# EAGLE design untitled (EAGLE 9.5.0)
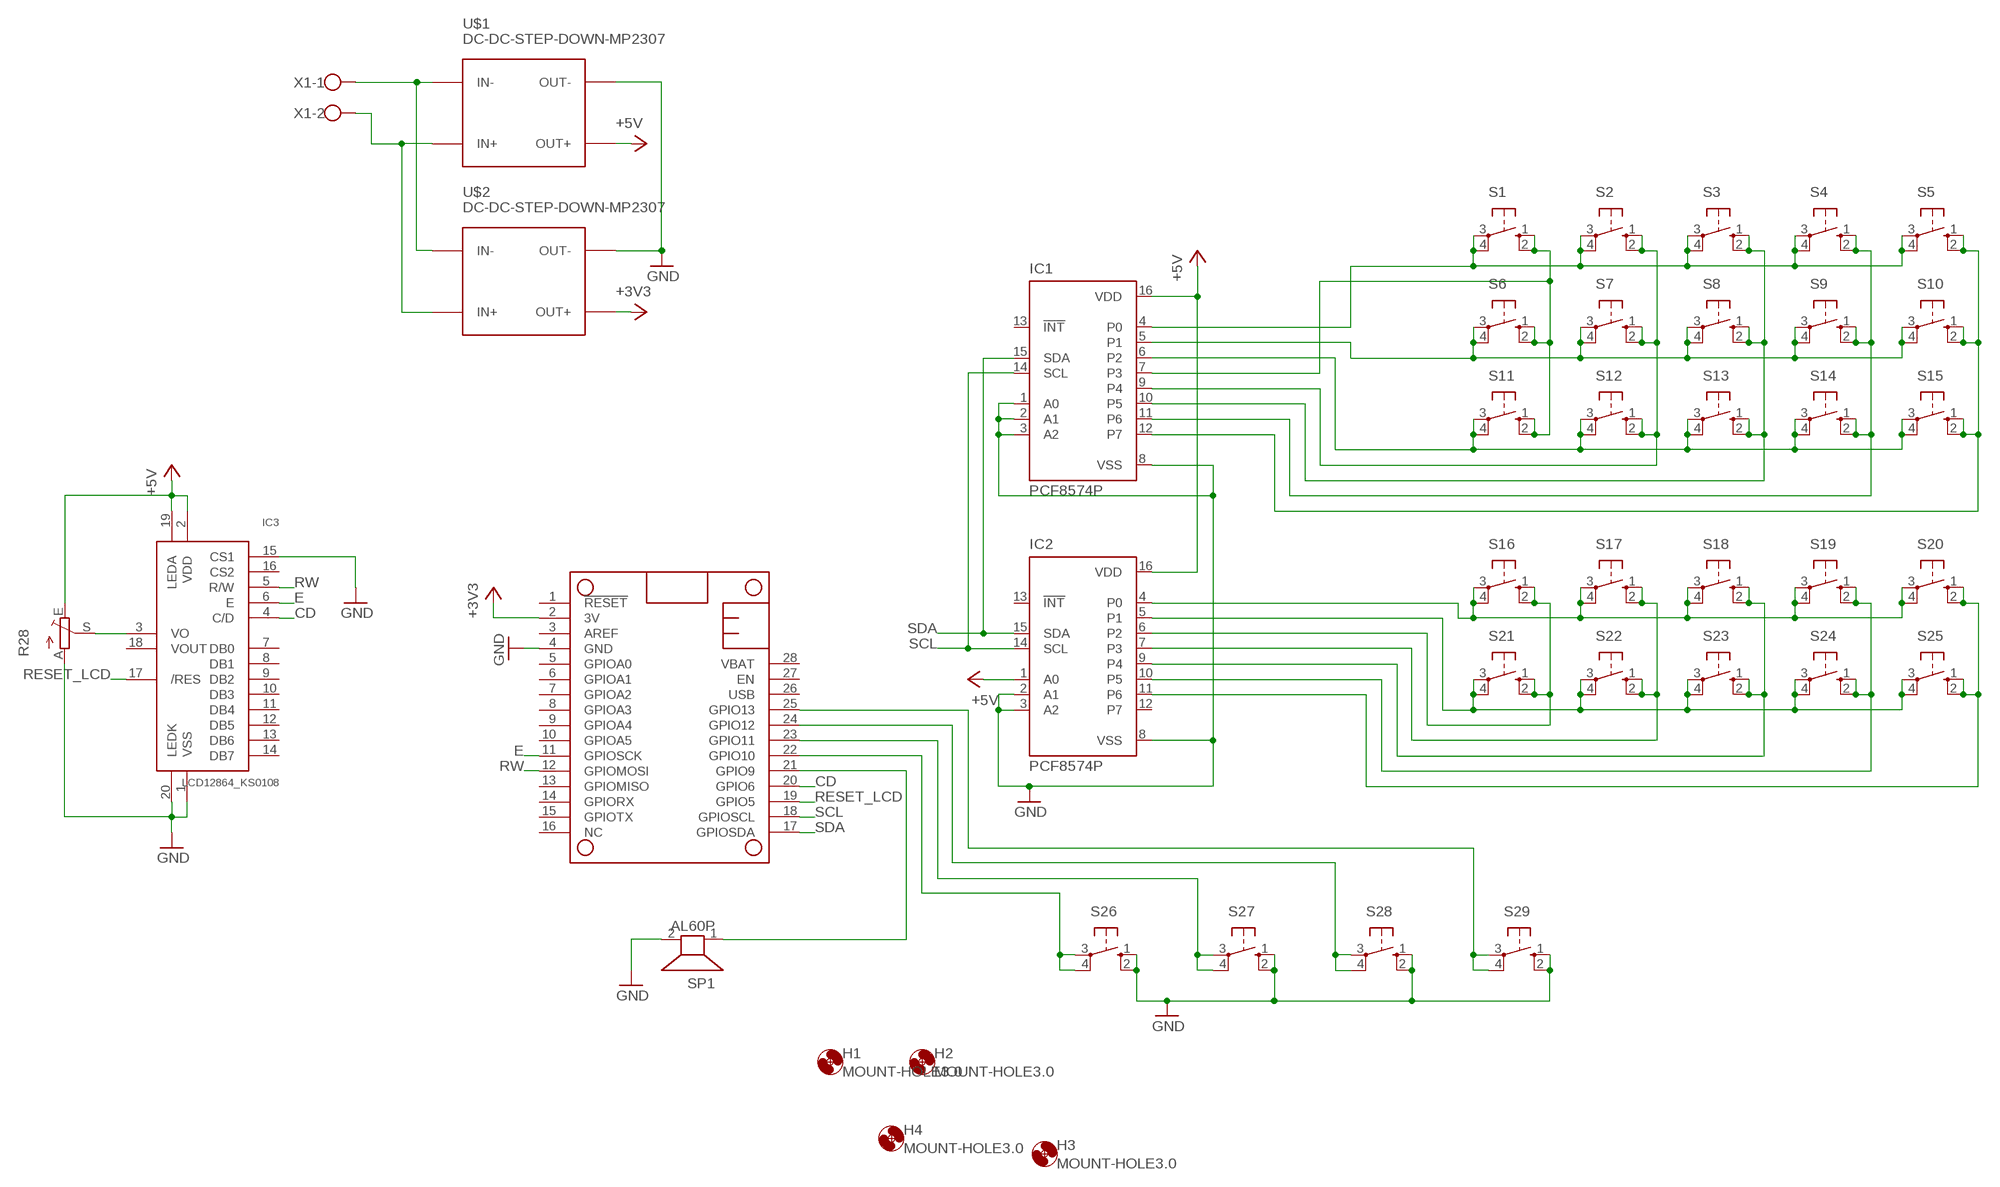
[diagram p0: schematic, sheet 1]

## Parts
H1  MOUNT-HOLE3.0  [3,0]
H2  MOUNT-HOLE3.0  [3,0]
H3  MOUNT-HOLE3.0  [3,0]
H4  MOUNT-HOLE3.0  [3,0]
IC1  PCF8574P  [DIL16]
IC2  PCF8574P  [DIL16]
IC3  LCD12864_KS0108  [RG12864]
MS1  FEATHERWING  [FEATHERWING]
R28  TRIM_EU-LI10  [LI10]
S1  10-XX  [B3F-10XX]
S2  10-XX  [B3F-10XX]
S3  10-XX  [B3F-10XX]
S4  10-XX  [B3F-10XX]
S5  10-XX  [B3F-10XX]
S6  10-XX  [B3F-10XX]
S7  10-XX  [B3F-10XX]
S8  10-XX  [B3F-10XX]
S9  10-XX  [B3F-10XX]
S10  10-XX  [B3F-10XX]
S11  10-XX  [B3F-10XX]
S12  10-XX  [B3F-10XX]
S13  10-XX  [B3F-10XX]
S14  10-XX  [B3F-10XX]
S15  10-XX  [B3F-10XX]
S16  10-XX  [B3F-10XX]
S17  10-XX  [B3F-10XX]
S18  10-XX  [B3F-10XX]
S19  10-XX  [B3F-10XX]
S20  10-XX  [B3F-10XX]
S21  10-XX  [B3F-10XX]
S22  10-XX  [B3F-10XX]
S23  10-XX  [B3F-10XX]
S24  10-XX  [B3F-10XX]
S25  10-XX  [B3F-10XX]
S26  10-XX  [B3F-10XX]
S27  10-XX  [B3F-10XX]
S28  10-XX  [B3F-10XX]
S29  10-XX  [B3F-10XX]
SP1  AL60P  [AL60P]
U$1  DC-DC-STEP-DOWN-MP2307  [DC-DC-STEP-DOWN-MP2307]
U$2  DC-DC-STEP-DOWN-MP2307  [DC-DC-STEP-DOWN-MP2307]
X1  W237-102  [W237-102]

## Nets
3V: MS1.2(3V) ; supply symbol labelled +3V3
+3V3: U$2.OUT+
+5V: IC1.16(VDD) IC2.1(A0) IC2.16(VDD) IC3.2(VDD) IC3.19(LEDA) R28.E U$1.OUT+
CD: IC3.4(C/D) MS1.20(GPIO6)
E: IC3.6(E) MS1.11(GPIOSCK)
GND: IC1.1(A0) IC1.2(A1) IC1.3(A2) IC1.8(VSS) IC2.2(A1) IC2.3(A2) IC2.8(VSS) IC3.1(VSS) IC3.15(CS1) IC3.20(LEDK) MS1.4(GND) R28.A S26.1(S) S26.2(S1) S27.1(S) S27.2(S1) S28.1(S) S28.2(S1) S29.1(S) S29.2(S1) SP1.2 U$1.OUT- U$2.OUT-
N$1: IC1.4(P0) S1.3(P) S1.4(P1) S2.3(P) S2.4(P1) S3.3(P) S3.4(P1) S4.3(P) S4.4(P1) S5.3(P) S5.4(P1)
N$3: IC1.5(P1) S6.3(P) S6.4(P1) S7.3(P) S7.4(P1) S8.3(P) S8.4(P1) S9.3(P) S9.4(P1) S10.3(P) S10.4(P1)
N$4: MS1.25(GPIO13) S29.3(P) S29.4(P1)
N$5: MS1.24(GPIO12) S28.3(P) S28.4(P1)
N$6: MS1.23(GPIO11) S27.3(P) S27.4(P1)
N$7: MS1.22(GPIO10) S26.3(P) S26.4(P1)
N$8: IC1.6(P2) S11.3(P) S11.4(P1) S12.3(P) S12.4(P1) S13.3(P) S13.4(P1) S14.3(P) S14.4(P1) S15.3(P) S15.4(P1)
N$9: IC1.7(P3) S1.1(S) S1.2(S1) S6.1(S) S6.2(S1) S11.1(S) S11.2(S1)
N$10: MS1.21(GPIO9) SP1.1
N$11: IC1.10(P5) S3.1(S) S3.2(S1) S8.1(S) S8.2(S1) S13.1(S) S13.2(S1)
N$12: IC1.11(P6) S4.1(S) S4.2(S1) S9.1(S) S9.2(S1) S14.1(S) S14.2(S1)
N$13: IC1.12(P7) S5.1(S) S5.2(S1) S10.1(S) S10.2(S1) S15.1(S) S15.2(S1)
N$16: U$1.IN- U$2.IN- X1.1
N$17: U$1.IN+ U$2.IN+ X1.2
N$21: IC1.9(P4) S2.1(S) S2.2(S1) S7.1(S) S7.2(S1) S12.1(S) S12.2(S1)
N$26: IC2.4(P0) S16.3(P) S16.4(P1) S17.3(P) S17.4(P1) S18.3(P) S18.4(P1) S19.3(P) S19.4(P1) S20.3(P) S20.4(P1)
N$28: IC2.7(P3) S17.1(S) S17.2(S1) S22.1(S) S22.2(S1)
N$29: IC2.5(P1) S21.3(P) S21.4(P1) S22.3(P) S22.4(P1) S23.3(P) S23.4(P1) S24.3(P) S24.4(P1) S25.3(P) S25.4(P1)
N$31: IC2.6(P2) S16.1(S) S16.2(S1) S21.1(S) S21.2(S1)
N$32: IC2.9(P4) S18.1(S) S18.2(S1) S23.1(S) S23.2(S1)
N$33: IC2.10(P5) S19.1(S) S19.2(S1) S24.1(S) S24.2(S1)
N$34: IC2.11(P6) S20.1(S) S20.2(S1) S25.1(S) S25.2(S1)
N$71: IC3.3(VO) R28.S
RESET_LCD: IC3.17(/RES) MS1.19(GPIO5)
RW: IC3.5(R/W) MS1.12(GPIOMOSI)
SCL: IC1.14(SCL) IC2.14(SCL) MS1.18(GPIOSCL)
SDA: IC1.15(SDA) IC2.15(SDA) MS1.17(GPIOSDA)
Unconnected: IC1.13(!INT) IC2.12(P7) IC2.13(!INT) IC3.7(DB0) IC3.8(DB1) IC3.9(DB2) IC3.10(DB3) IC3.11(DB4) IC3.12(DB5) IC3.13(DB6) IC3.14(DB7) IC3.16(CS2) IC3.18(VOUT) MS1.1(!RESET) MS1.3(AREF) MS1.5(GPIOA0) MS1.6(GPIOA1) MS1.7(GPIOA2) MS1.8(GPIOA3) MS1.9(GPIOA4) MS1.10(GPIOA5) MS1.13(GPIOMISO) MS1.14(GPIORX) MS1.15(GPIOTX) MS1.16(NC) MS1.26(USB) MS1.27(EN) MS1.28(VBAT)

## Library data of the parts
H1-H4 = holes:MOUNT-HOLE: MOUNTING HOLE with drill center marker
IC1 IC2 = micro-philips:PCF8574: I2C-Bus Remote 8-bit I/O expander http://www.semiconductors.philips.com/acrobat_download/datasheets/PCF8574_4.pdf
IC3 = DodoLcdR2:LCD12864_KS0108: LCD 128 x 64 controller KS0108
MS1 = adafruit:FEATHERWING
R28 = pot:TRIM_EU-: POTENTIOMETER
S1-S29 = switch-omron:10-XX: OMRON SWITCH; MPN: B3F-1000; OC_FARNELL: 176432; OC_NEWARK: 36M3542
SP1 = buzzer:AL60P: SPEAKER; OC_FARNELL: unknown; OC_NEWARK: unknown
U$1 U$2 = diy-modules:DC-DC-STEP-DOWN-MP2307: DC/DC Step-Down Regulator based on MP2307DN chip MP2307 datasheet available here: https://cdn-shop.adafruit.com/datasheets/MP2307_r1.9.pdf Click here to find device on ebay.com
X1 = con-wago-500:W237-102: WAGO SCREW CLAMP; MPN: 237-102; OC_FARNELL: unknown; OC_NEWARK: 70K9898

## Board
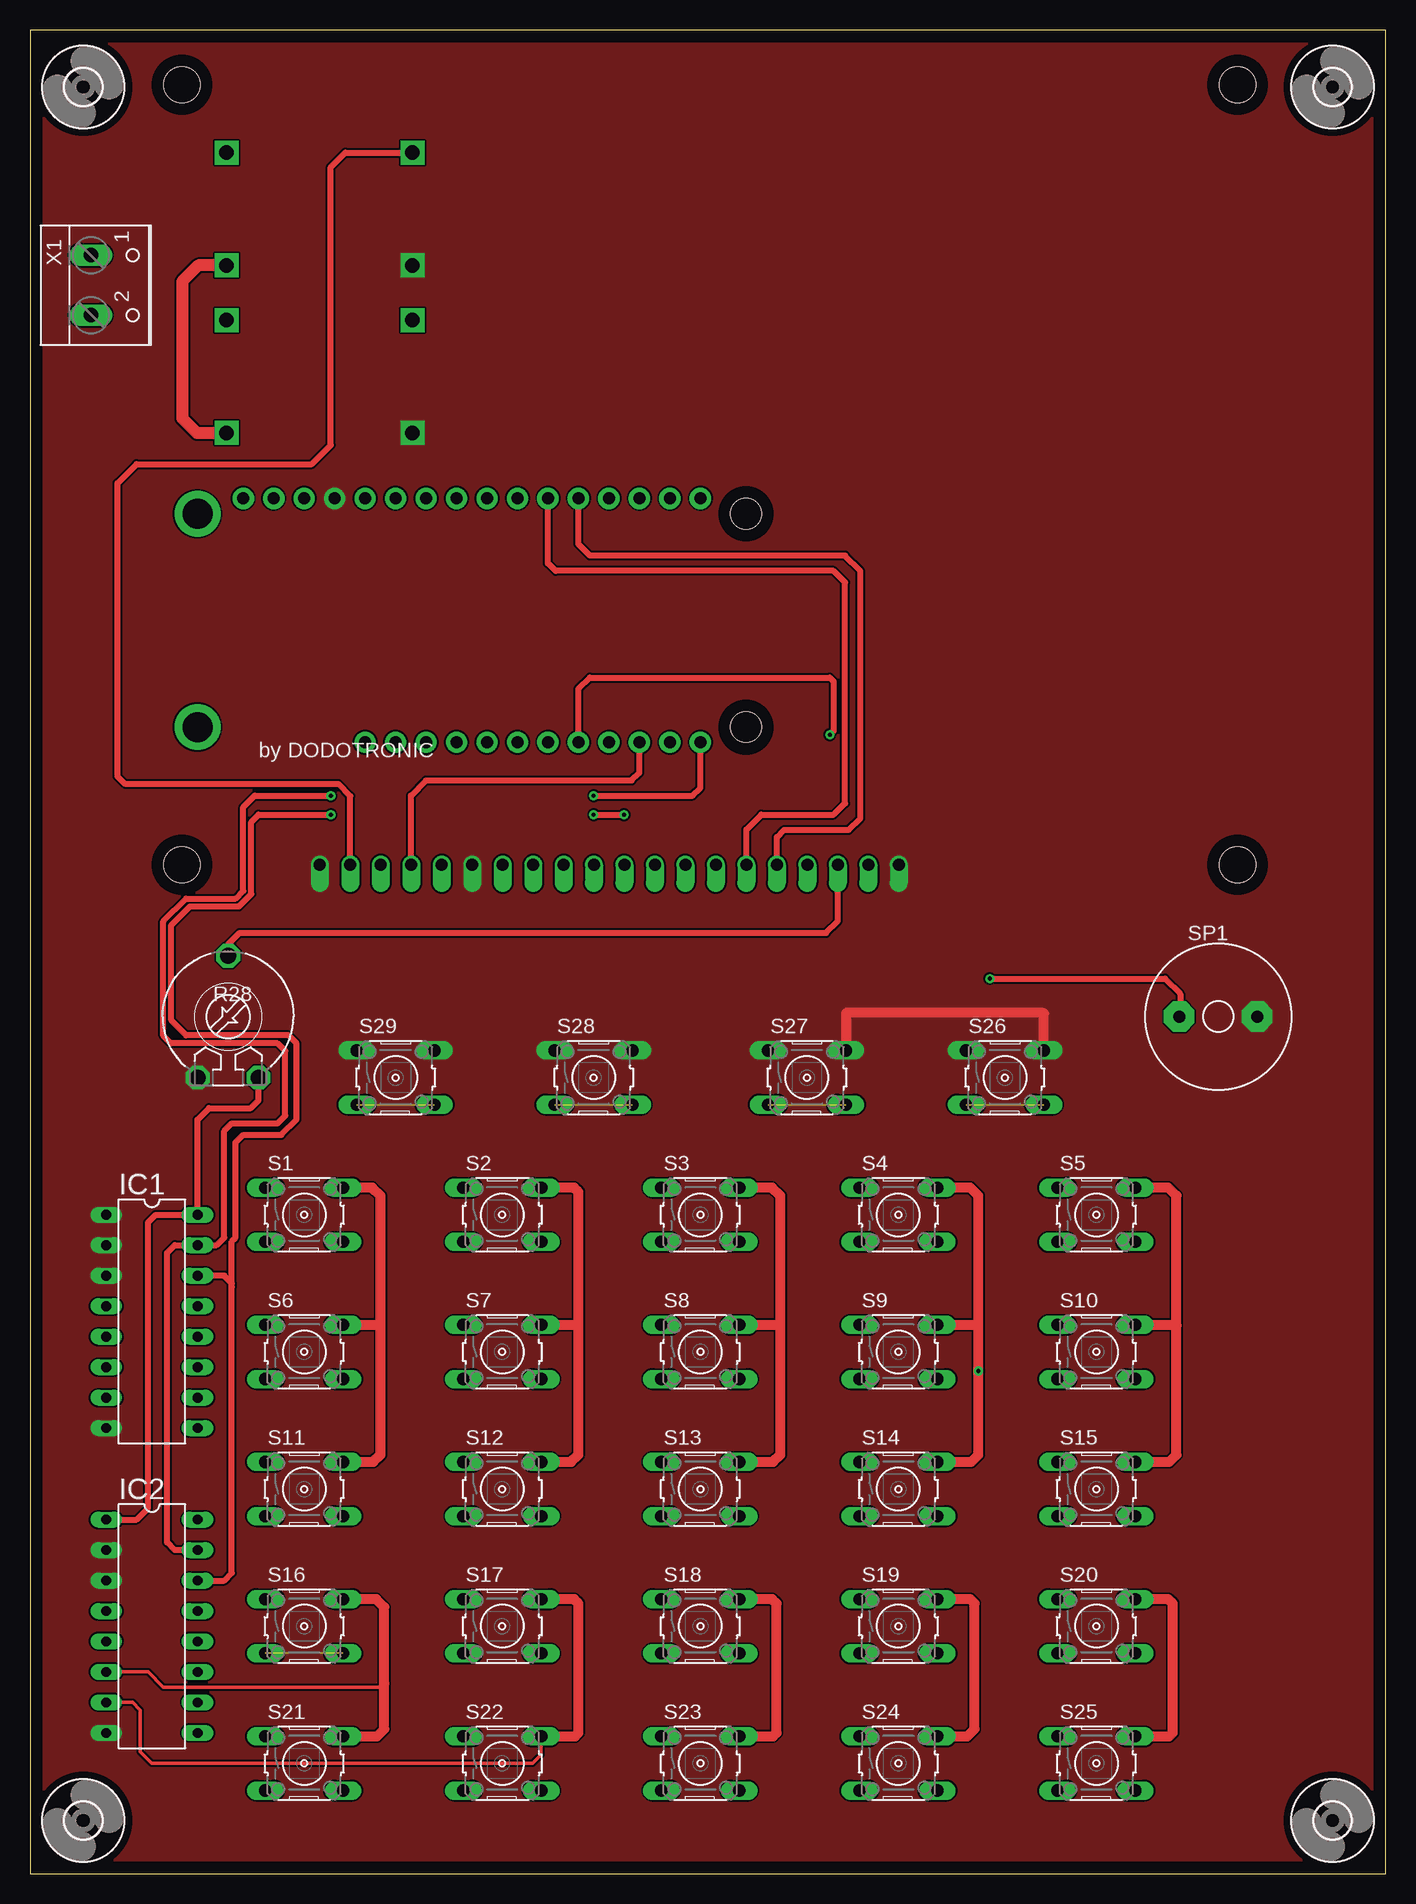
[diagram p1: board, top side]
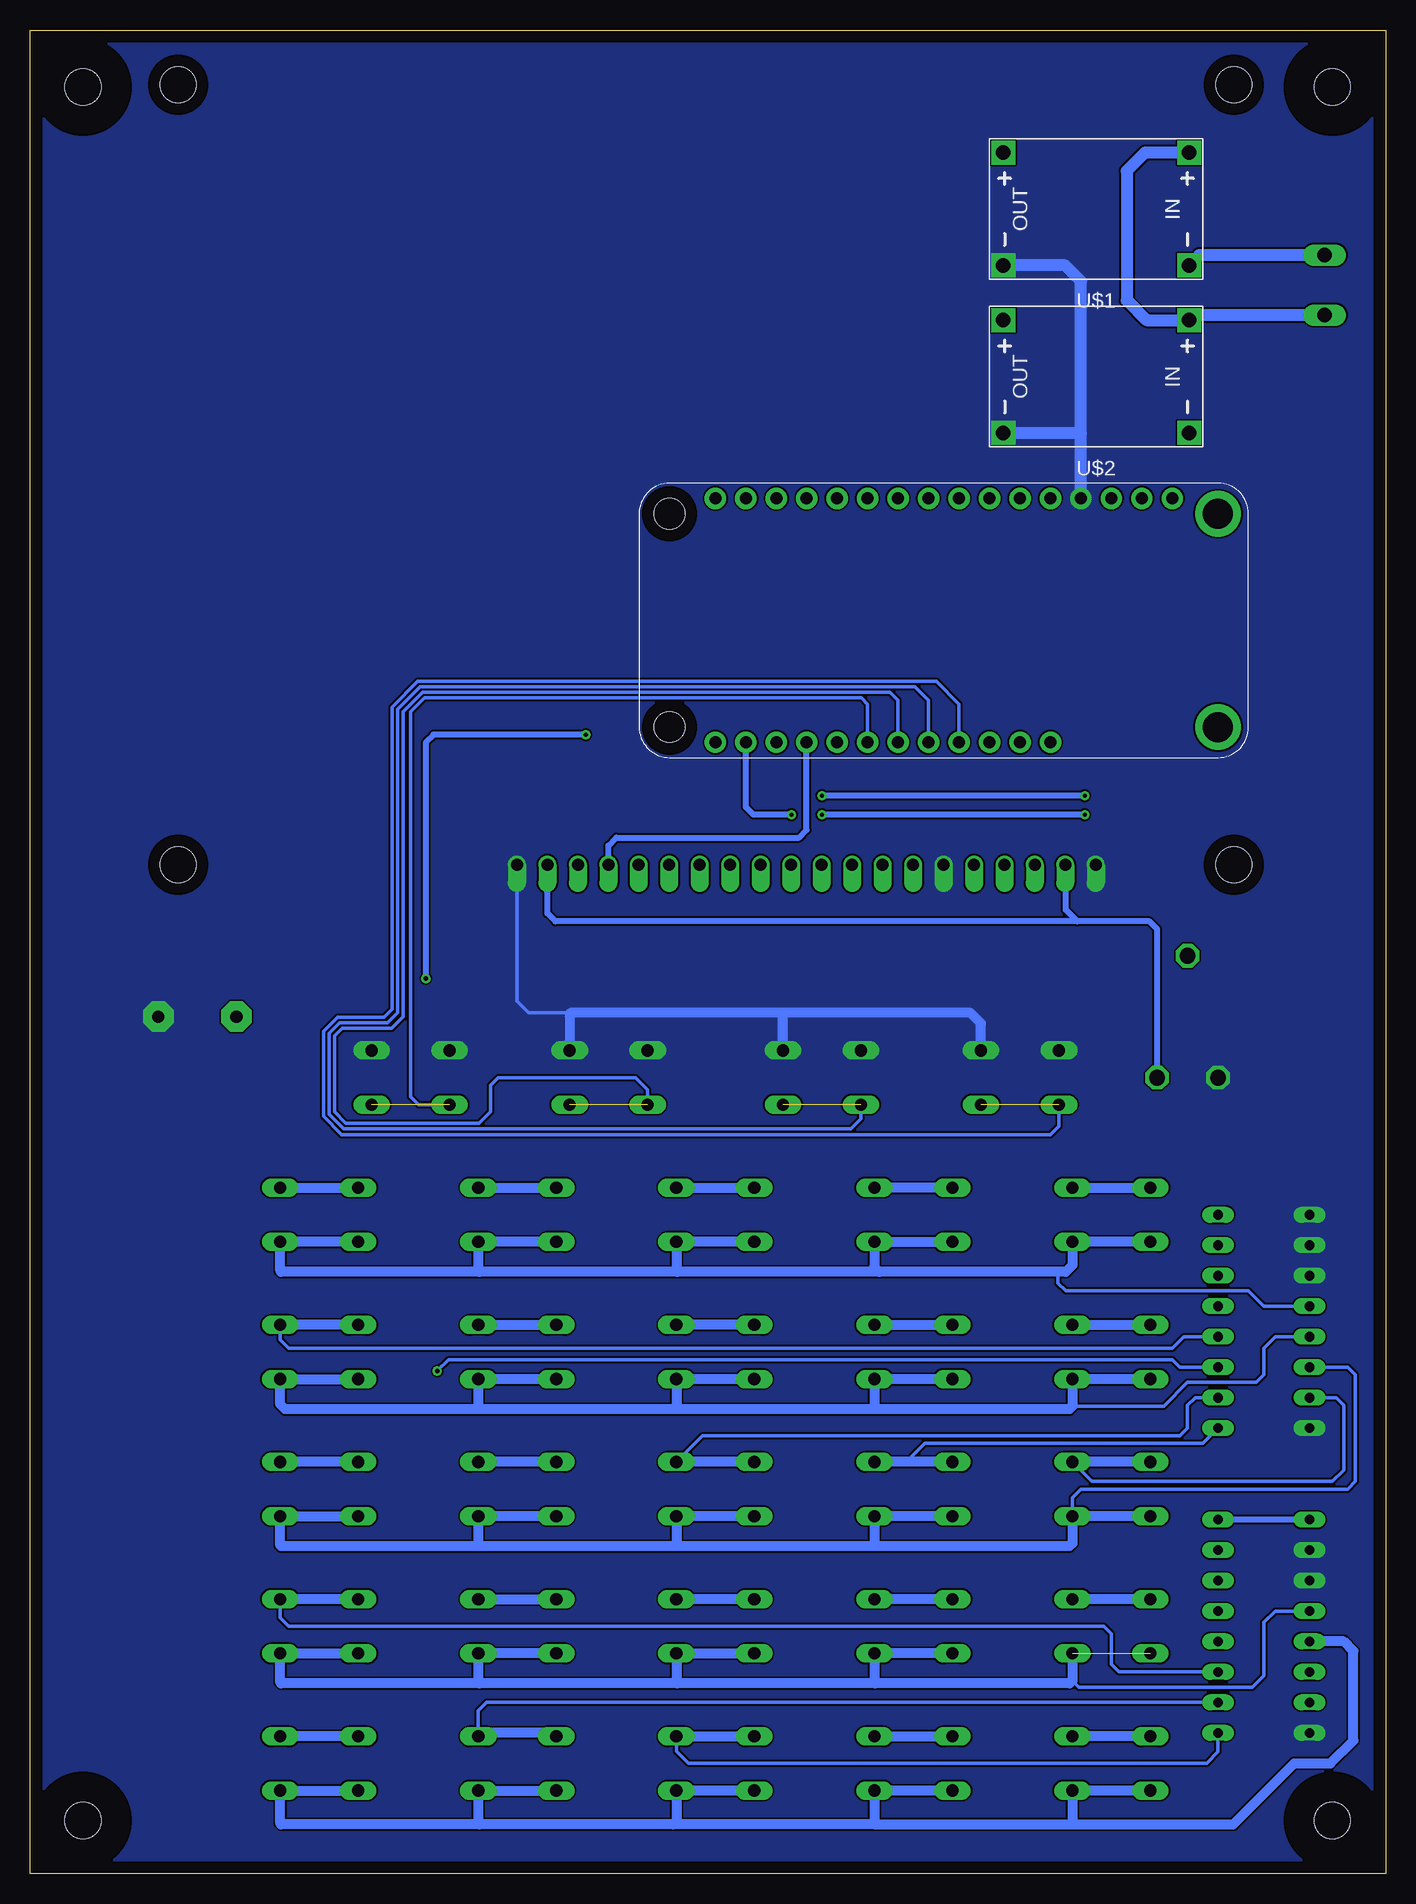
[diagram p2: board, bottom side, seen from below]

Size 113.01 x 153.66 mm. Coordinates in mm from the lower left corner, seen from the top.
Outline: 0,0 113.01,0 113.01,153.66 0,153.66 0,0
Copper layers (1*16): Top 0.035mm / dielectric 1.5mm / Bottom 0.035mm
Design rules "default": minimum track width 6mil, minimum drill 0.35mm, track to track 6mil, track to pad 6mil, pad to pad 6mil, via to via 6mil, smd to smd 6mil, copper to edge 40mil, drill to drill 6mil, minimum pad ring 10mil, minimum via ring 8mil, stop-mask expansion 4mil, vias tented up to drill 0mil, thermal gap 10mil

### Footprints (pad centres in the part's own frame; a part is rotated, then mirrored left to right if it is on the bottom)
3,0 = hole 3: 0,0
DIL16 = drill 0.813 long: 1 -8.89,-3.81; 2 -6.35,-3.81; 3 -3.81,-3.81; 4 -1.27,-3.81; 5 1.27,-3.81; 6 3.81,-3.81; 7 6.35,-3.81; 8 8.89,-3.81; 9 8.89,3.81; 10 6.35,3.81; 11 3.81,3.81; 12 1.27,3.81; 13 -1.27,3.81; 14 -3.81,3.81; 15 -6.35,3.81; 16 -8.89,3.81
RG12864 = drill 1 offset: 1 62.26,2.5; 2 59.72,2.5; 3 57.18,2.5; 4 54.64,2.5; 5 52.1,2.5; 6 49.56,2.5; 7 47.02,2.5; 8 44.48,2.5; 9 41.94,2.5; 10 39.4,2.5; 11 36.86,2.5; 12 34.32,2.5; 13 31.78,2.5; 14 29.24,2.5; 15 26.7,2.5; 16 24.16,2.5; 17 21.62,2.5; 18 19.08,2.5; 19 16.54,2.5; 20 14,2.5 | hole 3: 2.5,2.5; 90.5,2.5; 90.5,67.5; 2.5,67.5
FEATHERWING = drill 1 pad 1.778: 1 6.35,1.27; 2 8.89,1.27; 3 11.43,1.27; 4 13.97,1.27; 5 16.51,1.27; 6 19.05,1.27; 7 21.59,1.27; 8 24.13,1.27; 9 26.67,1.27; 10 29.21,1.27; 11 31.75,1.27; 12 34.29,1.27; 13 36.83,1.27; 14 39.37,1.27; 15 41.91,1.27; 16 44.45,1.27; 17 44.45,21.59; 18 41.91,21.59; 19 39.37,21.59; 20 36.83,21.59; 21 34.29,21.59; 22 31.75,21.59; 23 29.21,21.59; 24 26.67,21.59; 25 24.13,21.59; 26 21.59,21.59; 27 19.05,21.59; 28 16.51,21.59 | drill 2.5 pad 3.81: P$1 2.54,20.32; P$2 2.54,2.54 | hole 2.54: 48.26,20.32; 48.26,2.54
LI10 = drill 1.321 octagon: A -2.54,-5.08; E 2.54,-5.08; S 0,5.08
B3F-10XX = drill 1.016 long: 1 -3.251,2.261; 2 3.251,2.261; 3 -3.251,-2.261; 4 3.251,-2.261
AL60P = drill 1.016 pad 2.54 octagon: 1 -3.251,0; 2 3.251,0
DC-DC-STEP-DOWN-MP2307 = drill 1.2 pad 2 square: IN+ -7.747,-4.699; IN- -7.747,4.699; OUT+ 7.747,-4.699; OUT- 7.747,4.699
W237-102 = drill 1.194 long: 1 -2.5,-1.27; 2 2.5,-1.27

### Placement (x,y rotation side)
H1  4.45,4.45 0 top
H2  108.59,4.45 0 top
H3  4.45,148.91 0 top
H4  108.59,148.91 0 top
IC1  10.16,46.04 270 top
IC2  10.16,20.64 270 top
IC3  10.16,81.6 0 top
MS1  11.43,115.89 180 bottom
R28  16.51,71.44 0 top
S1  22.86,54.93 0 top
S2  39.37,54.93 0 top
S3  55.88,54.93 0 top
S4  72.39,54.93 0 top
S5  88.9,54.93 0 top
S6  22.86,43.5 0 top
S7  39.37,43.5 0 top
S8  55.88,43.5 0 top
S9  72.39,43.5 0 top
S10  88.9,43.5 0 top
S11  22.86,32.07 0 top
S12  39.37,32.07 0 top
S13  55.88,32.07 0 top
S14  72.39,32.07 0 top
S15  88.9,32.07 0 top
S16  22.86,20.64 0 top
S17  39.37,20.64 0 top
S18  55.88,20.64 0 top
S19  72.39,20.64 0 top
S20  88.9,20.64 0 top
S21  22.86,9.21 0 top
S22  39.37,9.21 0 top
S23  55.88,9.21 0 top
S24  72.39,9.21 0 top
S25  88.9,9.21 0 top
S26  81.28,66.36 0 top
S27  64.77,66.36 0 top
S28  46.99,66.36 0 top
S29  30.48,66.36 0 top
SP1  99.06,71.44 0 top
U$1  24.13,138.75 180 bottom
U$2  24.13,124.78 180 bottom
X1  6.35,132.4 270 top

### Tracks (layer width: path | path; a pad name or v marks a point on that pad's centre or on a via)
+5V
  Top 0.508: IC3.19 26.7,89.82 25.72,90.81 7.94,90.81 7.3,91.44 7.3,115.89 8.89,117.48 23.5,117.48 25.08,119.06 25.08,142.24 26.29,143.45 U$1.OUT+ | IC2.1 8.89,29.53 9.84,30.48 9.84,54.29 10.48,54.93 IC1.16 13.97,62.86 14.92,63.82 18.42,63.82 19.05,64.45 R28.E
  Bottom 0.508: R28.E 19.05,78.74 19.68,79.37 25.72,79.37 | 25.72,79.37 26.67,80.33 26.67,84.07 IC3.19 | 25.72,79.37 69.22,79.37 69.88,80.04 IC3.2 | IC2.1 IC2.16
CD
  Bottom 0.508: IC3.4 64.8,85.7 64.14,86.36 48.9,86.36 48.26,87 MS1.20
E
  Top 0.508: IC3.6 59.72,87.03 60.96,88.26 66.99,88.26 67.95,89.22 67.95,107.63 66.99,108.59 43.81,108.59 43.18,109.22 MS1.11
GND
  Top 0.813: S26.2 84.53,71.68 84.45,71.75 68.02,71.75 S27.2
  Bottom 0.305: IC3.1 72.42,72.74 71.44,71.75 67.95,71.75
  Bottom 0.813: S29.2 33.73,70.88 34.61,71.75 50.48,71.75 | S27.2 68.02,71.68 67.95,71.75 50.48,71.75 | S28.2 50.24,71.51 50.48,71.75
  Bottom 1.016: MS1.4 25.4,120.01 | 25.4,120.01 25.4,132.72 26.73,134.05 U$1.OUT- | U$2.OUT- 25.46,120.08 25.4,120.01
  pour Bottom (no thermals): 0,0 113.03,0 113.03,153.67 0,153.67
  pour Top (no thermals): 0,0 113.03,0 113.03,153.67 0,153.67
N$1
  Bottom 0.305: IC1.4 10.16,47.31 11.43,48.58 26.67,48.58 27.31,49.21 27.31,50.16
  Bottom 0.813: 42.23,50.16 27.31,50.16 26.67,50.16 26.11,50.72 S1.4 S1.3 | 42.23,50.16 59.06,50.16 | 59.06,50.16 75.56,50.16 | 75.56,50.16 92.08,50.16 92.15,50.24 S5.4 92.11,52.71 91.44,52.71 91.4,52.67 S5.3 | 75.56,50.16 75.64,50.24 S4.4 S4.3 | 59.06,50.16 59.13,50.24 S3.4 S3.3 | 42.23,50.16 42.62,50.56 S2.4 S2.3
N$3
  Bottom 0.305: IC1.5 9.21,44.77 10.16,43.81 10.16,41.59 10.79,40.96 16.51,40.96 18.49,38.98 26.11,38.98
  Bottom 0.813: 42.55,38.74 26.35,38.74 26.11,38.98 S6.4 S6.3 | 42.55,38.74 59.06,38.74 | 59.06,38.74 75.56,38.74 | 75.56,38.74 91.76,38.74 92.15,39.13 S10.4 S10.3 | 75.56,38.74 75.64,38.81 S9.4 S9.3 | 59.06,38.74 59.13,38.81 S8.4 S8.3 | 42.55,38.74 42.62,38.81 S7.4 S7.3
N$4  (1 unrouted)
  Bottom 0.305: S29.3 27.23,62.31 27.94,61.6 87.02,61.6 88.54,63.12 88.54,70.23 87.37,71.4 83.5,71.4 82.83,72.07 82.83,97.23 80.68,99.38 37.47,99.38 35.56,97.47 MS1.25
N$5  (1 unrouted)
  Bottom 0.305: S28.3 43.74,62.94 44.59,62.09 86.87,62.09 88.09,63.31 88.09,70.04 87.18,70.94 83.19,70.94 82.37,71.75 82.37,97.04 80.49,98.92 39.23,98.92 38.1,97.79 MS1.24
N$6  (1 unrouted)
  Bottom 0.305: S27.3 61.52,65.33 62.55,66.36 73.98,66.36 74.61,65.72 74.61,63.5 75.56,62.55 86.68,62.55 87.63,63.5 87.63,69.85 87,70.48 82.87,70.48 81.92,71.44 81.92,96.85 80.3,98.46 41.31,98.46 40.64,97.79 MS1.23
N$7  (1 unrouted)
  Bottom 0.305: S26.3 80.61,64.1 81.28,64.77 81.28,96.84 80.11,98.01 43.71,98.01 43.18,97.47 MS1.22
N$8
  Bottom 0.305: S11.4 26.11,29.84 26.11,31.36 25.4,32.07 3.18,32.07 2.54,32.7 2.54,41.59 3.18,42.23 IC1.6
  Bottom 0.813: S11.4 26.11,27.55 26.35,27.31 42.55,27.31 | 42.55,27.31 59.06,27.31 | 59.06,27.31 75.56,27.31 | 75.56,27.31 92.08,27.31 92.15,27.38 S15.4 S15.3 | 75.56,27.31 75.64,27.38 S14.4 S14.3 | 59.06,27.31 59.13,27.38 S13.4 S13.3 | 42.55,27.31 42.62,27.38 S12.4 S12.3 | S11.3 26.07,29.81 26.11,29.84
N$9
  Top 0.813: S11.2 28.61,34.33 29.21,34.92 29.21,45.72 | 29.21,45.72 29.21,56.51 28.54,57.19 S1.2 | S6.2 29.17,45.76 29.21,45.72
  Bottom 0.305: IC1.7 4.13,39.69 3.49,39.05 3.49,33.66 4.45,32.7 24.49,32.7 S11.2
  Bottom 0.813: S11.1 S11.2 | S6.2 S6.1 | S1.2 S1.1
N$10  (via drill 0.35)
  Top 0.508: MS1.21 45.72,98.74 46.67,99.7 66.68,99.7 66.99,99.38 66.99,95.25 v66.68,94.93 | v80.01,74.61 94.62,74.61 95.89,73.34 95.89,71.51 SP1.1
  Bottom 0.508: v66.68,94.93 79.38,94.93 80.01,94.3 v80.01,74.61
N$11
  Top 0.813: S13.2 61.95,34.33 62.55,34.92 62.55,45.72 | 62.55,45.72 62.55,56.51 61.87,57.19 S3.2 | S8.2 62.51,45.76 62.55,45.72
  Bottom 0.305: IC1.10 15.88,39.69 16.51,39.05 16.51,37.15 17.14,36.51 56.95,36.51 S13.2
  Bottom 0.813: S13.1 S13.2 | S8.1 S8.2 | S3.2 S3.1
N$12  (via drill 0.35)
  Top 0.813: S14.2 78.46,34.33 79.06,34.92 v79.06,41.91 79.06,45.72 | 79.06,45.72 79.06,56.51 78.38,57.19 S4.2 | S9.2 79.02,45.76 79.06,45.72
  Bottom 0.305: IC1.11 17.14,42.23 17.78,42.86 78.11,42.86 v79.06,41.91
  Bottom 0.813: S14.1 S14.2 | S9.2 S9.1 | S4.2 S4.1
N$13
  Top 0.813: S15.2 94.97,34.33 95.57,34.92 95.57,45.72 | 95.57,45.72 95.57,56.51 94.89,57.19 S5.2 | S10.2 95.53,45.76 95.57,45.72
  Bottom 0.305: IC1.12 16.83,44.77 17.78,43.81 91.44,43.81 92.15,44.53 S10.2
  Bottom 0.813: S15.1 S15.2 | S10.1 S10.2 | S5.2 S5.1
N$16
  Top 1.016: U$1.IN- 14.03,134.05 12.7,132.72 12.7,121.28 13.91,120.08 U$2.IN-
  Bottom 1.016: X1.1 15.53,134.9 U$1.IN-
N$17
  Bottom 1.016: X1.2 15.96,129.9 U$2.IN+ 19.94,129.48 21.59,131.13 21.59,141.92 20.07,143.45 U$1.IN+
N$21
  Top 0.813: S12.2 45.12,34.33 45.72,34.92 45.72,45.72 | 45.72,45.72 45.72,56.83 45.36,57.19 S2.2 | S7.2 45.68,45.76 45.72,45.72
  Bottom 0.305: IC1.9 15.24,35.88 38.42,35.88 40.01,34.29 42.58,34.29 S12.2
  Bottom 0.813: S12.1 42.55,34.33 42.58,34.29 | S7.2 S7.1 | S2.1 S2.2
N$26  (1 unrouted)
  Bottom 0.305: 26.11,16.12 25.55,15.56 11.11,15.56 10.16,16.51 10.16,20.96 9.21,21.91 IC2.4
  Bottom 0.813: S16.4 26.11,16.12 26.35,15.87 42.55,15.87 | 42.55,15.87 59.06,15.87 | 59.06,15.87 75.56,15.87 | 75.56,15.87 92.08,15.87 92.15,15.95 S20.4 S20.3 | 75.56,15.87 75.64,15.95 S19.4 S19.3 | 59.06,15.87 59.13,15.95 S18.4 S18.3 | 42.55,15.87 42.62,15.95 S17.4 S17.3
N$28
  Top 0.305: IC2.7 8.57,14.29 9.21,13.65 9.21,10.16 10.16,9.21 41.91,9.21 42.62,9.92 S22.2
  Top 0.813: S22.2 45.44,11.47 45.72,11.75 45.72,22.54 45.36,22.9 S17.2
  Bottom 0.813: S17.1 S17.2 | S22.2 S22.1
N$29
  Bottom 0.813: 26.35,4.13 26.11,4.37 S21.4 S21.3 | 42.55,4.13 26.35,4.13 | 42.55,4.13 59.37,4.13 | 59.37,4.13 75.56,4.13 | 75.56,4.13 92.08,4.13 92.15,4.2 S25.4 S25.3 | 75.56,4.13 75.64,4.2 S24.4 S24.3 | 59.37,4.13 59.13,4.37 S23.4 S23.3 | 42.55,4.13 42.62,4.2 S22.4 S22.3 | 26.35,4.13 12.7,4.13 7.62,9.21 4.6,9.21 2.69,11.11 2.69,18.57 3.49,19.37 IC2.5
N$31
  Top 0.305: IC2.6 9.84,16.83 11.11,15.56 29.21,15.56 29.53,15.87
  Top 0.813: S21.2 28.93,11.47 29.53,12.07 29.53,15.87 29.53,22.22 28.85,22.9 S16.2
  Bottom 0.813: S16.1 S16.2 | S21.1 S21.2
N$32
  Top 0.813: S23.2 61.95,11.47 62.23,11.75 62.23,22.54 61.87,22.9 S18.2
  Bottom 0.305: IC2.9 13.97,10.16 14.92,9.21 58.1,9.21 59.13,10.24 S23.2
  Bottom 0.813: S18.1 S18.2 | S23.2 S23.1
N$33
  Top 0.813: S24.2 78.14,11.47 78.74,12.07 78.74,22.54 78.38,22.9 S19.2
  Bottom 0.305: IC2.10 74.93,14.29 75.64,13.58 75.64,11.75 S24.2
  Bottom 0.813: S19.2 S19.1 | S24.1 69.42,11.75 75.64,11.75
N$34
  Top 0.813: S25.2 94.97,11.47 95.25,11.75 95.25,22.54 94.89,22.9 S20.2
  Bottom 0.305: IC2.11 22.22,16.83 22.86,17.46 22.86,20 23.5,20.64 91.44,20.64 92.15,21.35 92.15,22.86 S20.2
  Bottom 0.813: S20.1 92.11,22.9 92.15,22.86 | S25.1 S25.2
N$71
  Top 0.508: R28.S 16.51,77.47 17.46,78.42 66.36,78.42 67.34,79.4 IC3.3
RESET_LCD
  Top 0.508: IC3.17 31.78,89.82 31.75,89.85 33.02,91.12 50.17,91.12 50.8,91.76 MS1.19
RW
  Top 0.508: IC3.5 62.26,86.39 62.87,87 68.26,87 69.22,87.95 69.22,108.59 67.95,109.86 46.67,109.86 45.72,110.81 MS1.12
SCL  (via drill 0.35)
  Top 0.508: IC2.14 16.19,24.45 16.83,25.08 16.83,48.9 16.83,49.21 | 16.83,49.21 16.19,49.85 IC1.14 | 16.83,49.21 16.83,52.71 17.14,53.02 17.14,60.96 17.78,61.6 20.96,61.6 22.22,62.86 22.22,69.22 21.57,69.88 13.02,69.88 11.77,71.12 11.77,79.06 13.34,80.62 17.42,80.62 18.44,81.64 18.44,87.66 19.05,88.26 v25.08,88.26 | v46.99,88.26 v49.53,88.26
  Bottom 0.508: v25.08,88.26 v46.99,88.26 | v49.53,88.26 52.7,88.26 53.34,88.9 MS1.18
SDA  (via drill 0.35)
  Top 0.508: IC2.15 12.07,26.99 11.43,27.62 11.43,51.75 12.07,52.39 IC1.15 15.56,52.39 16.19,53.02 16.19,61.91 16.83,62.55 20.64,62.55 21.27,63.18 21.27,68.58 20.64,69.22 11.75,69.22 11.11,69.85 11.11,79.37 13.02,81.28 17.14,81.28 17.78,81.92 17.78,88.9 18.73,89.85 v25.08,89.85 | v46.99,89.85 55.25,89.85 55.88,90.49 MS1.17
  Bottom 0.508: v25.08,89.85 v46.99,89.85

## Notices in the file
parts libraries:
diy-modules: Released under the Creative Commons Attribution 4.0 International License: http://creativecommons.org/licenses/by/4.0
